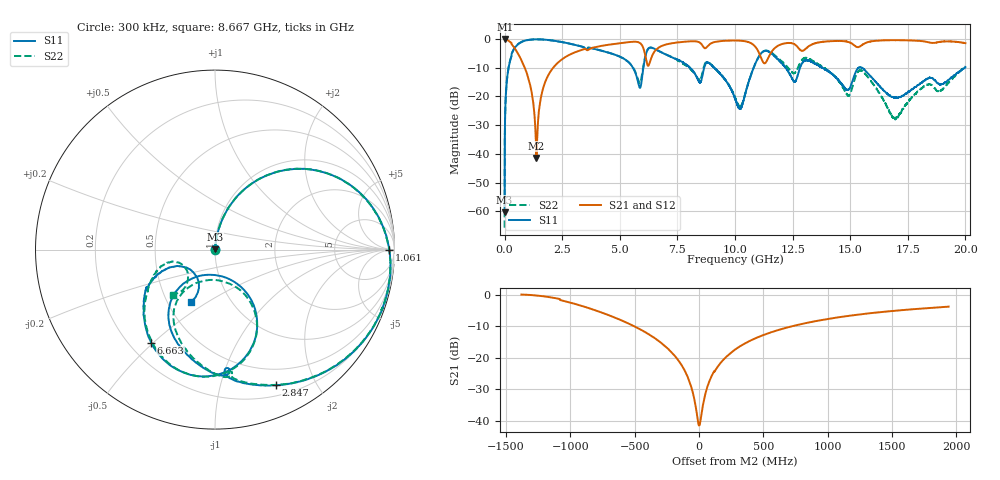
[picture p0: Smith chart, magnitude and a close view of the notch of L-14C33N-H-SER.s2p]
!{L-14C33N}
!Johanson Technology Inc.
!www.johansontechnology.com
!Test Board Conditions:
!Substrate Type  RO4350B
!Substrate Thickness  20 mil
!Substrate Dk  3.66
!TL Type: GCPW
!TL Trace Width  36 mil
!TL Gap  12 mil
!Electrode orientation  Horizontal
!DUT TOPOLOGY	SERIES
!Mounting Pad LxW  26x36 mil
! Created Sun Jun 20 13:04:36 2021
# hz S ma R 50
! 2 Port Network Data from SP1.SP block
! freq  magS11  angS11  magS21  angS21  magS12  angS12  magS22  angS22
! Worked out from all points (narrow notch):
!   20001 points, 300 kHz to 20 GHz, reference 50 ohm
!   highest |S21| = 0.00 dB at 2.3 MHz (marker M1); lowest = -41.4 dB at 1.382 GHz (marker M2)
!   notch at M2: 40.0 dB deep, 323 MHz wide at half that depth
!   lowest |S11| = -60.3 dB at 300 kHz (marker M3), VSWR 1.00, Z = 50.1 + j0.0634 ohm
!   |S11| at or under -10 dB: 9.105 GHz to 10.81 GHz (1.703 GHz wide, 17.1 % of centre); 13.8 GHz to 15.36 GHz (1.567 GHz wide, 10.7 % of centre); 15.52 GHz to 19.97 GHz (4.449 GHz wide, 25.1 % of centre)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
!   |S22| runs from -65.7 to -0.1 dB; largest |S21 - S12| = 0.014
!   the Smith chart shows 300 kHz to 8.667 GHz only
!   S11 on the Smith chart (normalised r, x): 300 kHz: 1.00, +0.00; 1.061 GHz: 67, -9; 2.847 GHz: 0.31, -1.50; 6.663 GHz: 0.29, -0.49; 8.667 GHz: 0.65, -0.42
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300000  0.0009641 41.0  0.9997 -0.1  0.9989 -0.0  0.0005183 49.9
2300000  0.004892 89.5  1 -0.3  0.9997 -0.3  0.004991 88.3
1.043e8  0.1989 74.9  0.9718 -12.6  0.9711 -12.7  0.1997 74.9
2.173e8  0.3881 63.1  0.9101 -25.4  0.9108 -25.3  0.3895 63.0
1.0613e9  0.9712 -0.2  0.1887 -87.4  0.189 -87.6  0.9716 -0.6
1.3823e9  0.9895 -15.0  0.008511 -16.3  0.008547 -16.3  0.9882 -15.2
1.8203e9  0.9712 -31.4  0.2034 56.3  0.2039 56.4  0.9694 -31.6
2.8473e9  0.8292 -65.8  0.5401 23.3  0.5415 23.2  0.8282 -65.4
3.3343e9  0.7436 -80.6  0.6458 8.6  0.6471 8.6  0.7441 -79.4
5.8583e9  0.1436 -102.6  0.8656 -66.0  0.8648 -66.0  0.1698 -96.2
6.2803e9  0.7012 -90.6  0.3678 -46.4  0.3687 -46.1  0.7048 -90.6
6.6633e9  0.6283 -124.5  0.7006 -41.6  0.7027 -41.5  0.6263 -123.8
6.6673e9  0.6266 -124.6  0.7028 -41.8  0.7043 -41.6  0.6254 -124.0
8.6673e9  0.3227 -115.1  0.7012 -91.7  0.7013 -91.6  0.3472 -133.4
1.00003e10  0.09226 -161.8  0.944 -112.9  0.9444 -112.8  0.09728 -176.4
1.12473e10  0.6148 -125.4  0.3845 -134.0  0.3861 -133.8  0.615 -137.7
1.25703e10  0.181 178.1  0.8198 -141.3  0.8192 -141.5  0.256 170.3
1.33343e10  0.3999 155.9  0.8041 -134.7  0.8008 -134.8  0.4261 141.7
1.49023e10  0.1301 154.9  0.8965 -172.5  0.8943 -172.4  0.1038 140.7
1.55343e10  0.3126 139.4  0.7998 -168.7  0.7941 -168.9  0.2747 126.9
1.66673e10  0.1059 138.0  0.9548 167.1  0.9559 167.4  0.05988 37.5
2e10  0.325 173.4  0.8496 103.2  0.8385 103.0  0.3359 -177.2
